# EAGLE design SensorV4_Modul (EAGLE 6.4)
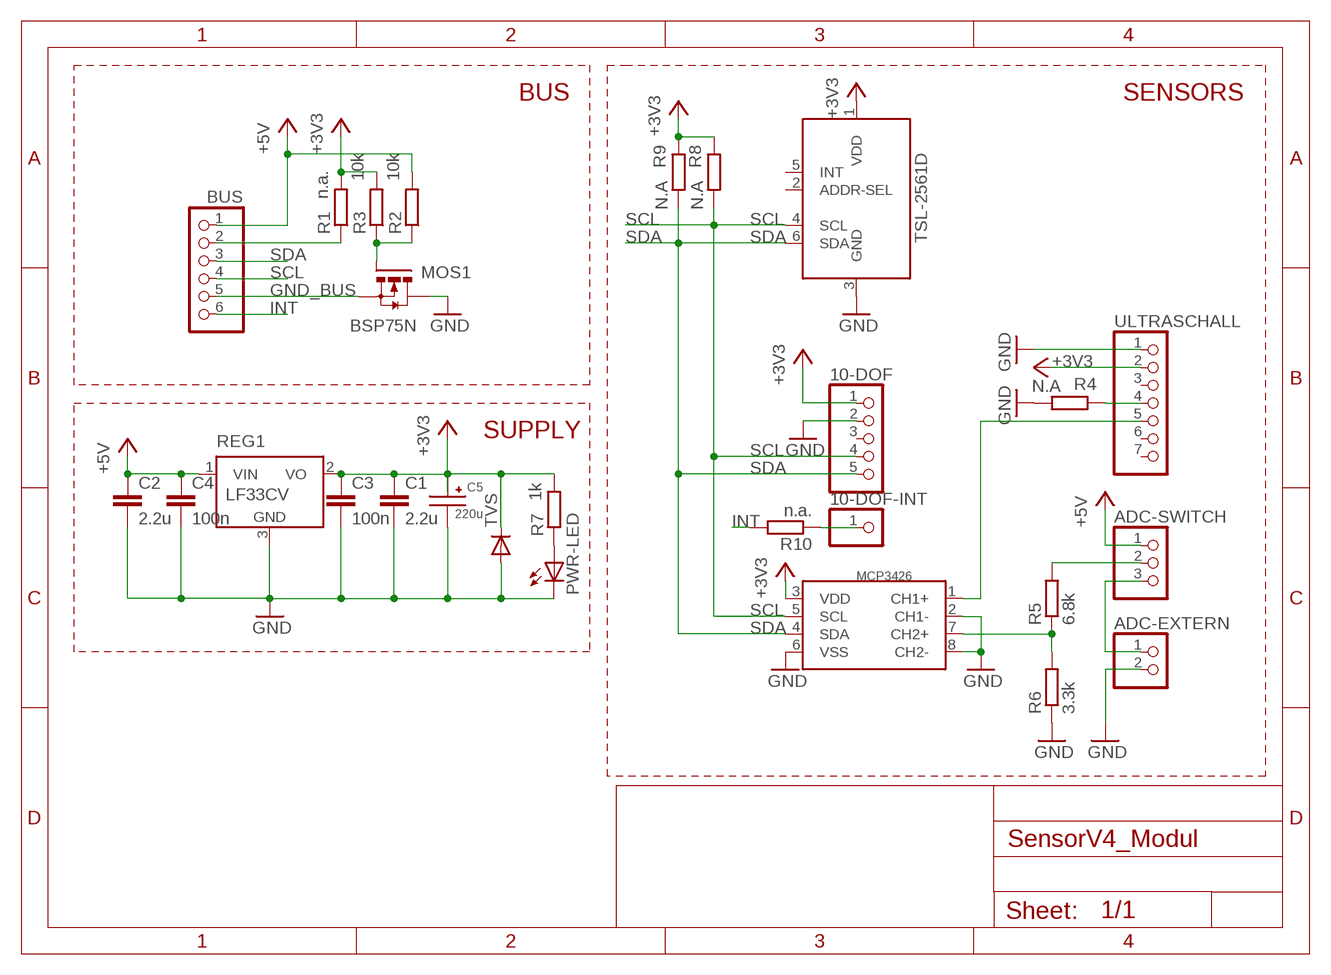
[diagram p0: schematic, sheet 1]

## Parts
10-DOF  PINHD-1X5  [1X05]
10-DOF-INT  PINHD-1X1  [1X01]
ADC-EXTERN  PINHD-1X2/90  [1X02/90]
ADC-SWITCH  PINHD-1X3  [1X03]
BUS  PINHD-1X6/90  [1X06/90]
C1  2.2u  C-EUC1206  [C1206]
C2  2.2u  C-EUC1206  [C1206]
C3  100n  C-EUC0805  [C0805]
C4  100n  C-EUC0805  [C0805]
C5  220u  C-SMC  [SMC]
MCP3426  MCP3426  [SOIC-8]
MOS1  BSP75N  N-HEXFET-2D_SOT232-  [SOT223]
PWR-LED  LEDCHIP-LED0805  [CHIP-LED0805]
R1  n.a.  R-EU_M0805  [M0805]
R2  10k  R-EU_M0805  [M0805]
R3  10k  R-EU_M0805  [M0805]
R4  N.A  R-EU_M0805  [M0805]
R5  6.8k  R-EU_M0805  [M0805]
R6  3.3k  R-EU_M0805  [M0805]
R7  1k  R-EU_M0805  [M0805]
R8  N.A  R-EU_M0805  [M0805]
R9  N.A  R-EU_M0805  [M0805]
R10  n.a.  R-EU_M0805  [M0805]
REG1  LF33CV  LM2936DT-3.3  [TO252]
TSL-2561D  TSL-2561D  [TMB6]
TVS  DIODE-SOD323-R  [SOD323-R]
ULTRASCHALL  PINHD-1X7  [1X07]

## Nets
+3V3: 10-DOF.1 C1.1 C3.1 C5.+ MCP3426.3(VDD) R1.2 R3.2 R7.2 R8.1 R9.1 REG1.2(VO) TSL-2561D.1(VDD) TVS.C ULTRASCHALL.2
+5V: ADC-SWITCH.1 BUS.1 C2.1 C4.1 R2.2 REG1.1(VIN)
GND: 10-DOF.2 ADC-EXTERN.2 C1.2 C2.2 C3.2 C4.2 C5.- MCP3426.2(CH1-) MCP3426.6(VSS) MCP3426.8(CH2-) MOS1.2(D) MOS1.4(D) PWR-LED.C R4.2 R6.1 REG1.3(GND) TSL-2561D.3(GND) TVS.A ULTRASCHALL.1
GND_BUS: BUS.5 MOS1.3(S)
INT: BUS.6 R10.2
N$1: BUS.2 R1.1
N$2: MOS1.1(G) R2.1 R3.1
N$3: R4.1 ULTRASCHALL.4
N$4: MCP3426.1(CH1+) ULTRASCHALL.5
N$5: MCP3426.7(CH2+) R5.1 R6.2
N$6: ADC-SWITCH.2 R5.2
N$7: ADC-EXTERN.1 ADC-SWITCH.3
N$8: PWR-LED.A R7.1
N$9: 10-DOF-INT.1 R10.1
SCL: 10-DOF.4 BUS.4 MCP3426.5(SCL) R8.2 TSL-2561D.4(SCL)
SDA: 10-DOF.5 BUS.3 MCP3426.4(SDA) R9.2 TSL-2561D.6(SDA)
Unconnected: 10-DOF.3 TSL-2561D.2(ADDR-SEL) TSL-2561D.5(INT) ULTRASCHALL.3 ULTRASCHALL.6 ULTRASCHALL.7

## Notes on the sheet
- BUS | SENSORS
- TSL-2561D
- SUPPLY

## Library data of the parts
10-DOF = pinhead:PINHD-1X5: PIN HEADER
10-DOF-INT = pinhead:PINHD-1X1: PIN HEADER
ADC-EXTERN = pinhead:PINHD-1X2: PIN HEADER
ADC-SWITCH = pinhead:PINHD-1X3: PIN HEADER
BUS = pinhead:PINHD-1X6: PIN HEADER
C1-C4 = resistor:C-EU: CAPACITOR, European symbol
C5 = Sensorbib:C-SMC
MCP3426 = Sensorbib:MCP3426; DESCRIPTION: MCP3426 von Farnell
MOS1 = transistor-power:N-HEXFET-2D_?-*: HEXFET® Power MOSFET 2 Drain connects http://www.irf.com/product-info/datasheets/data/irll014n.pdf
PWR-LED = led:LED: LED
R1-R10 = resistor:R-EU_: RESISTOR, European symbol
REG1 = national-semiconductor:LM2936?*: Ultra-Low Quiescent Current LDO Voltage Regulator Source: Data sheet; MPN: LM2936DT-3.3.; OC_FARNELL: 1286863; OC_NEWARK: 26M0361
TSL-2561D = Sensorbib:TSL-2561D
TVS = diode:DIODE-: DIODE
ULTRASCHALL = pinhead:PINHD-1X7: PIN HEADER

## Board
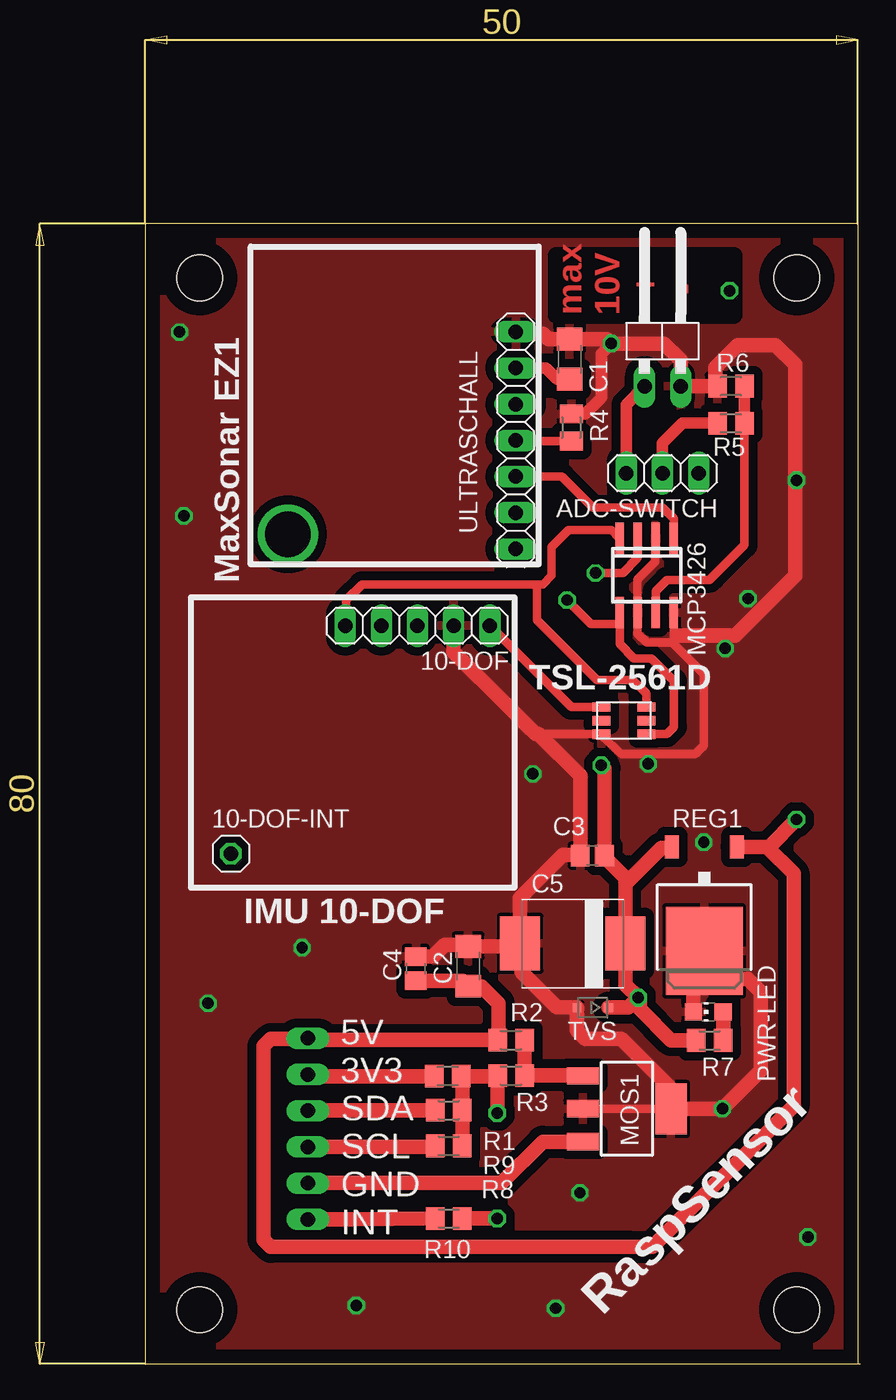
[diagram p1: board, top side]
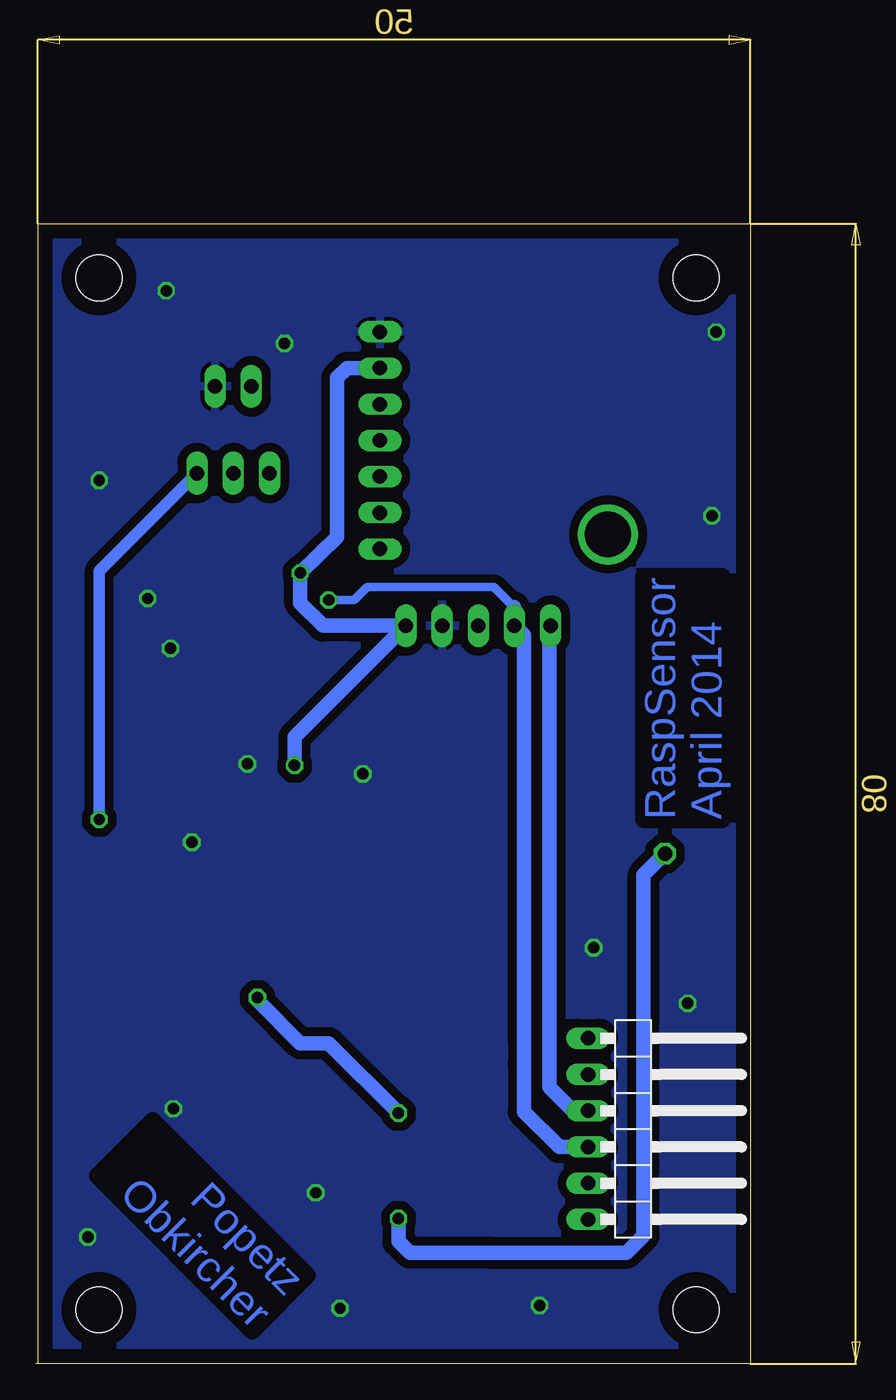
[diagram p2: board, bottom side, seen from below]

Size 57.87 x 93.2 mm. Coordinates in mm from the lower left corner, seen from the top.
Outline: 57.7,0 7.7,0 7.7,80 57.7,80 57.7,0
Outline: 57.7,0 57.87,0
Copper layers (1*16): Top 0.035mm / dielectric 1.5mm / Bottom 0.035mm
Design rules "default": minimum track width 10mil, minimum drill 24mil, track to track 8mil, track to pad 8mil, pad to pad 8mil, via to via 8mil, smd to smd 8mil, copper to edge 40mil, drill to drill 8mil, minimum pad ring 10mil, minimum via ring 8mil, stop-mask expansion 4mil, vias tented up to drill 0mil, thermal gap 10mil
Holes 3.2 mm at 11.51,76.2 11.51,3.81 53.42,76.2 53.42,3.81

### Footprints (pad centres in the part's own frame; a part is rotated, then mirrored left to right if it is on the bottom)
1X05 = drill 1.016 long: 1 -5.08,0; 2 -2.54,0; 3 0,0; 4 2.54,0; 5 5.08,0
1X01 = drill 1.016 octagon: 1 0,0
1X02/90 = drill 1.016 long: 1 -1.27,-3.81; 2 1.27,-3.81
1X03 = drill 1.016 long: 1 -2.54,0; 2 0,0; 3 2.54,0
1X06/90 = drill 1.016 long: 1 -6.35,-3.81; 2 -3.81,-3.81; 3 -1.27,-3.81; 4 1.27,-3.81; 5 3.81,-3.81; 6 6.35,-3.81
C1206 = smd 1.6 x 1.8: 1 -1.4,0; 2 1.4,0
C0805 = smd 1.3 x 1.5: 1 -0.85,0; 2 0.85,0
SMC = smd 2.8 x 3.8: + -3.7,0; - 3.7,0
SOIC-8 = smd 0.6 x 2.2: 1 -1.905,-2.6; 2 -0.635,-2.6; 3 0.635,-2.6; 4 1.905,-2.6; 5 1.905,2.6; 6 0.635,2.6; 7 -0.635,2.6; 8 -1.905,2.6
SOT223 = smd 1.219 x 2.235: 1 -2.311,-3.099; 2 0,-3.099; 3 2.311,-3.099 | smd 3.6 x 2.2: 4 0,3.099
CHIP-LED0805 = smd 1.2 x 1.2: A 0,-1.05; C 0,1.05
M0805 = smd 1.3 x 1.6: 1 -0.95,0; 2 0.95,0
TO252 = smd 1 x 1.6: 1 -2.28,-4.8; 2 2.28,-4.8 | smd 5.4 x 6.2: 3 0,2.5
TMB6 = smd 1.27 x 0.66: 1 -1.587,0.953; 2 -1.587,0; 3 -1.587,-0.953; 4 1.587,-0.953; 5 1.587,0; 6 1.587,0.953
SOD323-R = smd 0.6 x 0.6: A 1.1,0; C -1.1,0
1X07 = drill 1.016 long: 1 -7.62,0; 2 -5.08,0; 3 -2.54,0; 4 0,0; 5 2.54,0; 6 5.08,0; 7 7.62,0

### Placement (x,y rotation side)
10-DOF  26.8,51.8 180 top
10-DOF-INT  13.7,35.8 0 top
ADC-EXTERN  44,72.4 0 top
ADC-SWITCH  44,62.5 180 top
BUS  15.29,16.49 270 bottom
C1  37.48,70.5 90 top
C2  30.36,27.9 90 top
C3  39.07,35.67 180 top
C4  26.68,27.73 90 top
C5  37.7,29.5 180 top
MCP3426  42.88,55.32 180 top
MOS1  41.5,17.9 270 top
PWR-LED  47.2,24.7 90 top
R1  28.92,20.19 0 top
R2  33.37,22.72 180 top
R3  33.37,20.23 180 top
R4  37.6,65.7 90 top
R5  48.8,66 180 top
R6  48.8,68.6 0 top
R7  47.3,22.7 180 top
R8  29,15.3 180 top
R9  29,17.8 180 top
R10  29,10.2 180 top
REG1  46.93,31.48 180 top
TSL-2561D  41.29,45.14 0 top
TVS  39.1,25 180 top
ULTRASCHALL  33.7,64.8 270 top

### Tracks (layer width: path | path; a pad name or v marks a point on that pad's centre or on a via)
+3V3  (via drill 0.8)
  Top 0.61: TSL-2561D.1 37.59,46.09 10-DOF.1 | 32.38,20.19 R3.2 32.4,20.21 | R1.2 29.95,20.11 | MCP3426.3 42.25,56.55 41.2,55.5 v39.3,55.5
  Top 0.813: C1.1 36.58,69.1 35.8,69.88 ULTRASCHALL.2
  Top 1.016: 39.92,41.78 v39.7,42 39.92,41.78 | 32.38,20.19 R1.2 | 29.95,20.11 R9.1 R8.1 | 32.4,20.21 v32.4,17.6 | TVS.C 41.6,25 v42.3,25.7 | v42.3,25.7 41.4,26.6 C5.+ 41.4,33.7 41.6,33.9 | R7.2 44.6,22.7 42.4,24.9 42.4,25.6 v42.3,25.7 | 41.6,33.9 43.9,36.2 44.57,36.2 REG1.2 | 41.6,33.9 39.92,35.58 C3.1 39.92,41.78
  Bottom 0.61: 31.7,51.98 10-DOF.1
  Bottom 1.016: v39.7,42 39.7,43.98 10-DOF.1 35.6,51.8 37.7,51.8 39.3,53.4 v39.3,55.5 36.7,58 36.7,69.2 36.02,69.88 ULTRASCHALL.2 | v32.4,17.6 37.3,22.5 39.3,22.5 42.3,25.5 v42.3,25.7
+5V  (via drill 0.8)
  Top 0.61: 19.22,22.72 BUS.1 19.06,22.8 | 29.98,26.88 C2.1 | 32.5,22.8 R2.2 | REG1.1 51.32,36.28
  Top 1.016: 19.22,22.72 R2.2 | C4.1 29.98,26.88 | C2.1 31.3,26.5 32.5,25.3 32.5,22.8 | 51.32,36.28 53.2,34.4 53.2,18.1 43.3,8.2 41.9,8.2 16.5,8.2 16,8.7 16,22.3 16.5,22.8 19.06,22.8 | REG1.1 51.48,36.28 v53.4,38.2
  Bottom 0.813: v53.4,38.2 53.4,55.64 ADC-SWITCH.1
GND  (via drill 0.8)
  Top 0.61: R6.1 47.75,68.7 47.7,68.7 | 35.3,44.2 TSL-2561D.3 39.7,44.1 41.1,42.8 46.3,42.8 46.9,43.4 46.9,45.1 46.9,48.4 44.8,50.5 | 46,26.7 46.5,26.7 46.5,28.55 REG1.3 | MOS1.2 MOS1.4 | 44.8,50.5 44.8,51 | 44.8,51 44.8,52.7 MCP3426.8 | 44.8,50.5 44.7,50.6 42.9,50.6 42.25,51.26 MCP3426.6 42.25,55.05 43.5,56.3 43.5,57.91 MCP3426.2 | 45,51.1 44.9,51.1 44.8,51 | 30.26,29.4 C2.2
  Top 0.813: R4.2 38.55,66.65 39.7,67.8 39.7,70.9 v40.4,71.6
  Top 1.016: R6.1 ADC-EXTERN.2 45.27,70.43 44.1,71.6 v40.4,71.6 40.1,71.9 C1.2 36,71.9 35.6,72.3 33.82,72.3 ULTRASCHALL.1 | 10-DOF.2 29.34,49.96 33.1,46.2 34.5,44.8 35.1,44.2 35.3,44.2 38.22,41.28 C3.2 38.19,35.7 37,35.7 34,32.7 C5.- | 47.7,68.7 47.7,69.9 49.3,71.5 51.9,71.5 53.3,70.1 53.3,55.3 49.1,51.1 45,51.1 | C4.2 27.88,28.58 28.7,29.4 30.26,29.4 | C5.- 34.1,29.4 34.1,27.5 36.6,25 TVS.A 38,23.4 38.6,22.8 41.1,22.8 44.5,19.4 44.5,18 MOS1.4 46.6,17.9 v48.2,17.9 50.9,20.6 50.9,26.1 50,27 46.2,27 46.15,26.95 PWR-LED.C 46.15,28.2 REG1.3 | C2.2 33.8,29.3 C5.-
  other vias: 50,53.7 43,42.1 48.4,50.2 34.9,41.4 18.7,29.2 12.1,25.3 38.2,12 54.2,8.9 22.5,4.1 36.5,3.9 53.4,62 48.7,75.3 10.4,59.5 10.1,72.4 46.9,36.6
  pour Bottom (isolate 0.61): 8.2,79.5 57.3,79.5 57.3,0.4 8.2,0.4
  pour Top (isolate 0.61): 8.4,0.7 57,0.7 57,79.4 8.3,79.4 8.3,0.7
GND_BUS
  Top 0.61: BUS.5 19.12,12.7
  Top 1.016: 19.12,12.7 32.7,12.7 35.59,15.59 MOS1.3
INT
  Top 1.016: BUS.6 22.19,10.14 R10.2
N$1
  Top 0.61: BUS.2 19.21,20.19
  Top 1.016: 19.21,20.19 R1.1
N$2
  Top 0.61: MOS1.1 38.38,20.23
  Top 1.016: 38.38,20.23 R3.1 R2.1
N$3
  Top 0.61: R4.1 33.75,64.75 ULTRASCHALL.4
N$4
  Top 0.61: ULTRASCHALL.5 36.94,62.26 39.1,60.1 44,60.1 44.8,59.3 44.8,58.5 44.8,57.94 MCP3426.1
N$5
  Top 0.61: R5.1 49.75,57.45 47.5,55.2 47.3,55 44.3,55 43.52,54.22 MCP3426.7
  Top 0.813: R6.2 R5.1
N$6
  Top 0.813: R5.2 45.4,66 44,64.6 ADC-SWITCH.2
N$7
  Top 0.813: ADC-SWITCH.3 41.46,67.32 ADC-EXTERN.1
N$8
  Top 1.016: R7.1 PWR-LED.A
N$9  (via drill 0.8)
  Top 1.016: R10.1 v32.4,10.2
  Bottom 1.016: v32.4,10.2 32.4,8.6 31.6,7.8 26,7.8 16.4,7.8 15.2,9 15.2,34.3 10-DOF-INT.1
N$10  (via drill 3.2)
  other vias: 17.7,58.2
SCL  (via drill 0.8)
  Top 0.61: 43.1,49.5 43.2,49.5 | 43.2,49.5 43.1,49.5 | 43.1,49.5 42,49.5 41,50.5 41,51.9 40.98,51.92 | R8.2 27.97,15.22 | MCP3426.5 40.98,51.92 | 40.98,51.92 38.98,51.92 v37.3,53.6 | TSL-2561D.4 44.29,44.19 44.8,44.7 44.8,47.9 43.2,49.5
  Top 1.016: 27.97,15.22 BUS.4
  Bottom 0.61: v37.3,53.6 35.5,53.6 34.6,54.5 25.7,54.5 24.3,53.1 | 24.3,51.84 10-DOF.4
  Bottom 1.016: BUS.4 21.12,15.22 23.6,17.7 23.6,21.1 23.6,22.8 23.6,51.14 10-DOF.4 | 24.3,53.1 24.3,51.84
SDA
  Top 0.61: 35.3,54.7 22.9,54.7 21.8,53.6 21.8,51.88 10-DOF.5 | BUS.3 19.14,17.8 | TSL-2561D.6 42.88,47.02 41.9,48 39.4,48 35.2,52.2 35.2,54.6 35.3,54.7 | 35.3,54.7 35.6,54.7 36.2,55.3 36.2,57.3 37.4,58.5 40.4,58.5 MCP3426.4
  Top 1.016: 19.14,17.8 R9.2
  Bottom 0.61: 10-DOF.5 21.8,51.72
  Bottom 1.016: 21.8,51.72 21.8,49.3 21.8,19.4 20.16,17.76 BUS.3

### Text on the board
Top: max / 10V / + / -
Bottom: RaspSensor / April 2014 | Popetz / Obkircher
tPlace: MaxSonar EZ1 | TSL-2561D | IMU 10-DOF | 5V / 3V3 / SDA / SCL / GND / INT | RaspSensor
